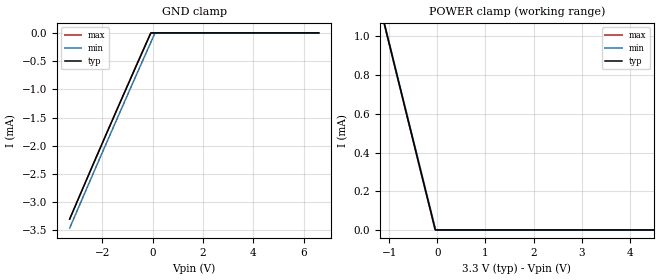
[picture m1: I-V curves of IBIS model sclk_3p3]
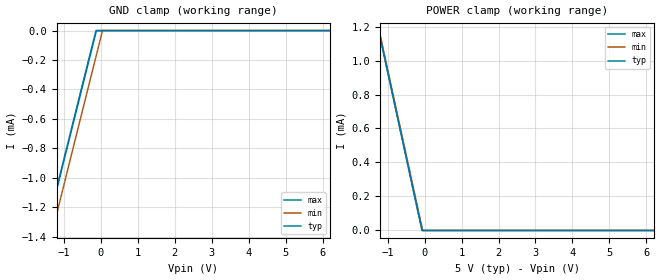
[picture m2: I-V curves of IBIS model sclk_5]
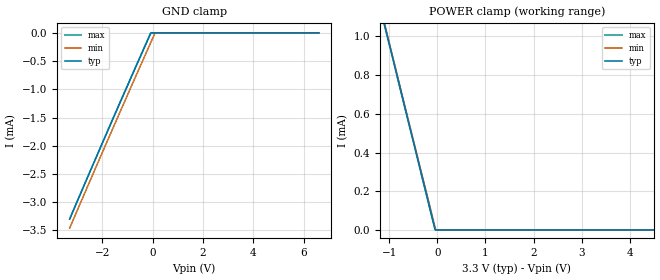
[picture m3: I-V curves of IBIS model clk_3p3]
|Texas Instruments Incorporated
| 24-Bit A/D Conv with 2-Channel Diff Input Multiplexer
| Marketing part#   Digital Voltage Range   Package-type   #pins
| ADS1222IPWR   2.7V  - 5.5V   TSSOP   14
| ADS1222IPWRG4   2.7V  - 5.5V   TSSOP   14
| ADS1222IPWT   2.7V  - 5.5V   TSSOP   14
| ADS1222IPWTG4   2.7V  - 5.5V   TSSOP   14
[IBIS Ver]   3.2
[File name]   ads1222.ibs
|SIMDE Ver   V2.2 - 201009 - RHL4 - Build 424
[File Rev]   1.0
[Date]   8/29/2011
[Source]
| Texas Instruments Incorporated.
| Analog-eLab Design Center, HPA
| 12500 TI Blvd
| Dallas, TX -75243
| e-mail: elab_scm_ibis@list.ti.com
[Notes]   Revision History:
| Rev 1.0: 8/29/2011
| - Initial version of the model
| - Model generated from simulations in SPECTRE
| - Model matched to SPICE simulation
| - C_comp although listed in numerical order of value are
|   obtained from varying PVT conditions. For PVT conditions for
|   each specific value refer the buffer description under
|   respective [Model]. IBIS model user is responsible for using
|   appropriate C_comp to simulate for Signal Integrity.
| - Model names with a trailing _3p3 contains the model for
|   3.3V [3.0V and 3.6V]. Model names with a trailing _5 contains
|   the model for 5.0V [4.5V and 5.5V].
|*  EXCEPTION:   *
|*  - For model sclk_* and clk_*, there is a small leakage current   *
|*   in the GND clamp I-V Table MIN corner because of a diode (D0)   *
|*   connected to the PAD.   *
|*  - For model bufen_*, there will be a leakage current in the POWER   *
|*   clamp I-V Table because of the pulldown on pad.   *
|*  - For model mux_tempen_*, there will be a small leakage current   *
|*   in the GND clamp I-V Table MIN corner because of a diode (D0)   *
|*   connected to pad.   *
[Disclaimer]
| This model is designed as an aid for customers of Texas Instruments.
| TI and its licensors and suppliers make no warranties, either expressed
| or implied, with respect to this  model, including the warranties of
| merchantability or fitness for a particular purpose. The model is
| provided solely on an "as is" basis. The entire risk as to its quality
| and performance is with the customer.
[Copyright]
 (C) Copyright 2011 Texas Instruments Incorporated.All rights reserved.
|   ADS1222PW
[Component]   ADS1222PW
[Manufacturer]   TI
[Package]   |14 TSSOP  -  PW package
|   typ   min   max
R_pkg   0.25163   0.21790   0.29401
L_pkg   2.25409nH   1.79858nH   3.08983nH
C_pkg   0.084903pF   0.07297pF   0.09772pF
[Pin]  signal_name   model_name   R_pin   L_pin   C_pin
1   VDD   POWER   0.13941   2.29201nH  0.17735pF
2   SCLK   SCLK   0.25190   2.09600nH  0.08550pF
3   CLK   CLK   0.21790   1.79858nH  0.07297pF
4   _DRDY/DOUT   DRDY_DOUT   0.22131   1.82860nH  0.07447pF
5   MUX   MUX_TEMPEN   0.24402   2.02821nH  0.08323pF
6   TEMPEN   MUX_TEMPEN   0.26325   2.19912nH  0.08898pF
7   BUFEN   BUFEN   0.28152   2.96670nH  0.09290pF
8   AINP2   TERM   0.29401   3.08983nH  0.09772pF
9   AINN2   TERM   0.27212   2.29468nH  0.09448pF
10   AINP1   TERM   0.23745   1.98620nH  0.08249pF
11   AINN1   TERM   0.21852   1.82055nH  0.07342pF
12   GND   GND   0.21915   1.82484nH  0.07330pF
13   VREFN   TERM   0.24785   2.07668nH  0.08338pF
14   VREFP   TERM   0.26976   2.86392nH  0.08930pF
1000   THERMAL_PAD   NC   0.00002   0.00103nH  1.04012pF
|   Model Selectors
[Model Selector] SCLK
sclk_3p3   3.3V digital input
sclk_5   5.0V digital input
[Model Selector] CLK
clk_3p3   3.3V digital input
clk_5   5.0V digital input
[Model Selector] BUFEN
bufen_3p3  3.3V digital input
bufen_5   5.0V digital input
[Model Selector] MUX_TEMPEN
mux_tempen_3p3  3.3V digital input
mux_tempen_5   5.0V digital input
[Model Selector] DRDY_DOUT
drdy_dout_3p3   3.3V digital output
drdy_dout_5   5.0V digital output
[Model Selector] TERM
term_3-3V  3.3V nominal termination
term_5-0V  5.0V nominal termination
[Model] term_3-3V
Model_type Terminator
C_comp   1.0e-20F  1.0e-20F  1.0e-20F
|   typ   min   max
[Voltage Range]   3.3V   3.0V   3.6V
[POWER Clamp Reference]   3.3V   3.0V   3.6V
[GND Clamp Reference]   0V   0V   0V
|Ambient Temperature   25   85   -40
|Junction Temperature
[Temperature Range]   25   85   -40
[Model] term_5-0V
Model_type Terminator
C_comp   1.0e-20F  1.0e-20F  1.0e-20F
|   typ   min   max
[Voltage Range]   5.0V   4.5V   5.5V
[POWER Clamp Reference]   5.0V   4.5V   5.5V
[GND Clamp Reference]   0V   0V   0V
|Ambient Temperature   25   85   -40
|Junction Temperature
[Temperature Range]   25   85   -40
| Models and submodels in the file (12): sclk_3p3 (Input), sclk_5 (Input), clk_3p3 (Input), clk_5 (Input), bufen_3p3 (Input), bufen_5 (Input), mux_tempen_3p3 (Input), mux_tempen_5 (Input), drdy_dout_3p3 (Output), drdy_dout_5 (Output), term_3-3V (Terminator), term_5-0V (Terminator)
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|   sclk_3p3 Model
[Model]   sclk_3p3
Model_type   Input
Vinl = 0.66
Vinh = 2.64
|   typ   min   max
|   (nom PVT)   (fast PVT)   (slow PVT)
|C_comp from frequency sweep method (F= 5MHz)
|Average
C_comp   2.052e-15   1.706e-15   2.457e-15
|C_comp from LC tank measurement(L=1nH)
|Average
|resonant Frequency(Hz)   1.000e+12   1.000e+12   1.000e+12
|C_comp   2.536e-17   2.536e-17   2.536e-17
[Model spec]
Vinl   0.66   0.6   0.72
Vinh   2.64   2.4   2.88
| Where nom  PVT is Nominal Process, 3.3V, 25C
|   Fast PVT is Strong Process,  3.6V, -40C
|   Slow PVT is Weak Process,   3V, 85C
[Voltage Range]   3.3   3   3.6
|Ambient Temperature   25   85   -40
|Junction Temperature
[Temperature Range]   25   85   -40
[Power Clamp Reference]   3.3   3   3.6
[GND Clamp Reference]   0   0   0
[GND Clamp]
|   Voltage   I(typ)   I(min)   I(max)
-3.3V     -3.299mA   -3.46mA    -3.299mA
-1.756V   -1.703mA   -1.867mA   -1.698mA
-81.6mV   -10.64uA   -174.8uA   -3.025uA
93mV      0A         0A         0A
6.6V      0A         0A         0A
[POWER Clamp]
|   Voltage   I(typ)   I(min)   I(max)
-3.3V     3.297mA    3.298mA    3.297mA
-1.136V   1.098mA    1.104mA    1.094mA
-825mV    784.3uA    790.6uA    780uA
-49.2mV   6.178uA    14.35uA    1.715uA
-42mV     1.155uA    7.161uA    0A
-30mV     0A         0A         0A
6.6V      0A         0A         0A
|   sclk_5 Model
[Model]   sclk_5
Model_type   Input
Vinl = 1
Vinh = 4
|   typ   min   max
|   (nom PVT)   (fast PVT)   (slow PVT)
|C_comp from frequency sweep method (F= 5MHz)
|Average
C_comp   2.384e-15   1.992e-15   2.857e-15
|C_comp from LC tank measurement(L=1nH)
|Average
|resonant Frequency(Hz)   1.000e+12   1.000e+12   1.000e+12
|C_comp   2.536e-17   2.536e-17   2.536e-17
[Model spec]
Vinl   1   0.9   1.1
Vinh   4   3.6   4.4
| Where nom  PVT is Nominal Process, 5V, 25C
|   Fast PVT is Strong Process,  5.5V, -40C
|   Slow PVT is Weak Process,   4.5V, 85C
[Voltage Range]   5   4.5   5.5
|Ambient Temperature   25   85   -40
|Junction Temperature
[Temperature Range]   25   85   -40
[Power Clamp Reference]   5   4.5   5.5
[GND Clamp Reference]   0   0   0
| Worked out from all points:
|   GND clamp passes 1 mA (typ) near -1.12 V on its own axis
|   POWER clamp passes 1 mA (typ) near -1.06 V on its own axis
[GND Clamp]
|   Voltage   I(typ)   I(min)   I(max)
-5V       -4.998mA   -5.159mA   -4.998mA
-1.728V   -1.621mA   -1.785mA   -1.609mA
-1.25V    -1.136mA   -1.301mA   -1.124mA
-226mV    -105.9uA   -270.6uA   -93.46uA
-138mV    -17.71uA   -182.5uA   -5.421uA
-127mV    -6.705uA   -171.5uA   0A
-115mV    0A         -159.5uA   0A
40mV      0A         0A         0A
10V       0A         0A         0A
[POWER Clamp]
|   Voltage   I(typ)   I(min)   I(max)
-5V       4.996mA    4.997mA    4.996mA
-1.247V   1.185mA    1.195mA    1.179mA
-1.106V   1.043mA    1.053mA    1.037mA
-72mV     6.562uA    19.92uA    290.4nA
-54.5mV   0A         2.47uA     0A
-45.5mV   0A         0A         0A
10V       0A         0A         0A
|   clk_3p3 Model
[Model]   clk_3p3
Model_type   Input
Vinl = 0.66
Vinh = 2.64
|   typ   min   max
|   (nom PVT)   (fast PVT)   (slow PVT)
|C_comp from frequency sweep method (F= 8MHz)
|Average
C_comp   8.016e-16   6.665e-16   9.597e-16
|C_comp from LC tank measurement(L=1nH)
|Average
|Resonant Frequency(Hz)   1.000e+12   1.000e+12   1.000e+12
|C_comp   2.536e-17   2.536e-17   2.536e-17
[Model spec]
Vinl   0.66   0.6   0.72
Vinh   2.64   2.4   2.88
| Where nom  PVT is Nominal Process, 3.3V, 25C
|   Fast PVT is Strong Process,  3.6V, -40C
|   Slow PVT is Weak Process,   3V, 85C
[Voltage Range]   3.3   3   3.6
|Ambient Temperature   25   85   -40
|Junction Temperature
[Temperature Range]   25   85   -40
[Power Clamp Reference]   3.3   3   3.6
[GND Clamp Reference]   0   0   0
[GND Clamp]
|   Voltage   I(typ)   I(min)   I(max)
-3.3V     -3.299mA   -3.46mA    -3.299mA
-1.756V   -1.703mA   -1.867mA   -1.698mA
-81.6mV   -10.64uA   -174.8uA   -3.025uA
93mV      0A         0A         0A
6.6V      0A         0A         0A
[POWER Clamp]
|   Voltage   I(typ)   I(min)   I(max)
-3.3V     3.297mA    3.298mA    3.297mA
-1.136V   1.098mA    1.104mA    1.094mA
-825mV    784.3uA    790.6uA    780uA
-49.2mV   6.178uA    14.35uA    1.715uA
-42mV     1.155uA    7.161uA    0A
-30mV     0A         0A         0A
6.6V      0A         0A         0A
